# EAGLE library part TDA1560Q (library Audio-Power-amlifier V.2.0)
The TDA1560Q is an integrated Bridge-Tied Load (BTL) class-H high power amplifier. In a load of 8 Ω , the output power is 40 W typical at a THD of 10%.
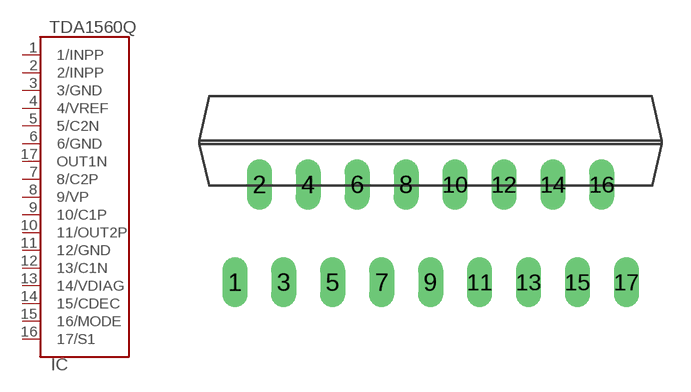
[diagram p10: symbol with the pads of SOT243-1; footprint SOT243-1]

Designator prefix IC

## TDA1560Q  [SOT243-1]
1  1/INPP  in
2  2/INPP  in
3  3/GND  pwr
4  4/VREF
5  5/C2N
6  6/GND  pwr
7  8/C2P
8  9/VP  pwr
9  10/C1P
10  11/OUT2P  out
11  12/GND  pwr
12  13/C1N
13  14/VDIAG  out
14  15/CDEC
15  16/MODE  in
16  17/S1  in
17  OUT1N  out

## Footprint SOT243-1 (pad centres in mm)
DBS17P: plastic DIL-bent-SIL power package; 17 leads (lead length 7.7 mm)
drill 0.8 long: 1 -10.16,-5.08; 2 -8.89,0; 3 -7.62,-5.08; 4 -6.35,0; 5 -5.08,-5.08; 6 -3.81,0; 7 -2.54,-5.08; 8 -1.27,0; 9 0,-5.08; 10 1.27,0; 11 2.54,-5.08; 12 3.81,0; 13 5.08,-5.08; 14 6.35,0; 15 7.62,-5.08; 16 8.89,0; 17 10.17,-5.08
